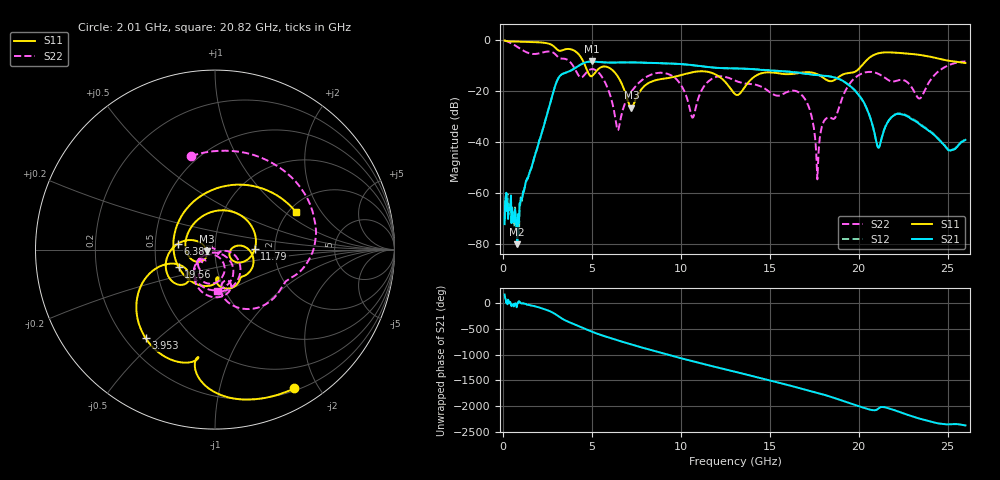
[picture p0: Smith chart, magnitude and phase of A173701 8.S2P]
!  2-Port S-parameters saved by WinCal
! VAR MeasName=S-Parameters (CALIBRATED_DATA) read from VNA (N5245A)
! VAR MeasDate=2017-6-7 10:28:54
! VAR NAME=A173701 8
! VAR FILENAME=A173701 8.S2P
! VAR DATE=2017-6-7 10:28:54
! VAR PHYS_PORTS=1,2
# Hz S DB R 50
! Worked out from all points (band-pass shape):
!   801 points, 100 MHz to 26 GHz, reference 50 ohm
!   highest |S21| = -8.52 dB at 5.021 GHz (marker M1); lowest = -80.0 dB at 812.2 MHz (marker M2)
!   |S21| within 3 dB of the highest: 3.965 GHz to 14.15 GHz (10.19 GHz wide, 112 % of centre)
!   lowest |S11| = -26.6 dB at 7.223 GHz (marker M3), VSWR 1.10, Z = 45.6 - j0.912 ohm
!   |S11| at or under -10 dB: 4.619 GHz to 20.19 GHz (15.57 GHz wide, 126 % of centre)
!   |S22| runs from -54.6 to -0.3 dB; largest |S21 - S12| = 0.0046
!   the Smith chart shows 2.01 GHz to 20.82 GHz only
!   S11 on the Smith chart (normalised r, x): 2.01 GHz: 0.23, -1.70; 3.953 GHz: 0.28, -0.46; 6.381 GHz: 0.66, +0.04; 11.79 GHz: 1.57, +0.02; 19.56 GHz: 0.65, -0.14; 20.82 GHz: 2.16, +1.22
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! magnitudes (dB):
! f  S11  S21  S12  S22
! 100 MHz  -0.3  -72.1  -70.3  -0.3
! 812.2 MHz  -0.8  -80.0  -80.7  -2.8
! 2.01 GHz  -1.0  -40.5  -40.5  -5.4
! 3.079 GHz  -4.0  -15.6  -15.6  -6.6
! 3.953 GHz  -4.0  -11.6  -11.5  -10.3
! 4.438 GHz  -7.4  -9.5  -9.5  -14.7
! 5.021 GHz  -14.2  -8.5  -8.5  -11.5
! 6.381 GHz  -13.6  -8.9  -8.9  -33.3
! 7.223 GHz  -26.6  -8.9  -8.9  -20.3
! 8.744 GHz  -15.6  -9.1  -9.2  -13.0
! 10.65 GHz  -12.7  -9.9  -10.0  -30.5
! 11.79 GHz  -13.1  -10.9  -10.9  -15.1
! 13.05 GHz  -21.2  -11.2  -11.2  -16.0
! 16.58 GHz  -13.1  -12.9  -12.8  -20.4
! 17.39 GHz  -12.8  -13.7  -13.5  -30.9
! 17.71 GHz  -13.6  -13.9  -13.8  -49.8
! 19.56 GHz  -13.0  -18.3  -18.3  -16.6
! 20.82 GHz  -6.1  -34.4  -34.5  -12.7
! 21.14 GHz  -5.3  -42.1  -42.1  -13.5
! 21.69 GHz  -4.9  -31.6  -31.5  -15.9
! 23.44 GHz  -6.0  -33.1  -32.8  -23.0
! 26 GHz  -9.1  -39.2  -39.0  -8.6
